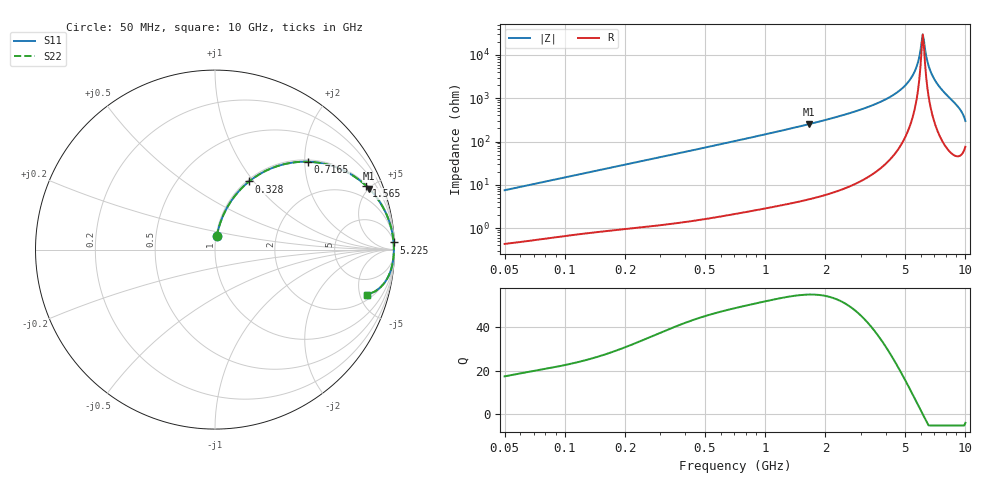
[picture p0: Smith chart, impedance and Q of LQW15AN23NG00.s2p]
!Murata Part Number: LQW15AN23NG00
!These Parameters are Measured in Series Mode Connection
!  o--[Z]--o
!Port1  Port2
!  o-------o
!Freq. Start=50[MHz] Stop=10[GHz], 401[Steps]
# Hz S RI R 50
!Freq.(Hz)	S 11(Real)	S 11(Imag)	S 21(Real)	S 21(Imag)	S 12(Real)	S 12(Imag)	S 22(Real)	S 22(Imag)
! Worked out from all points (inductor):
!   401 points, 50 MHz to 10 GHz, reference 50 ohm
!   read as one part in series: L = 23.7 nH near 51.34 MHz
!   highest Q = 54.6 at 1.651 GHz (marker M1), where L = 24.2 nH
!   self-resonance near 6.126 GHz
!   S11 on the Smith chart (normalised r, x): 50 MHz: 1.01, +0.15; 328 MHz: 1.02, +0.95; 716.5 MHz: 1.04, +2.08; 1.565 GHz: 1.09, +4.73; 5.225 GHz: 5, +50; 10 GHz: 2.51, -5.76
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5e7  0.00977 0.0737  0.9902 -0.0737  0.9902 -0.0737  0.00977 0.0737
1.214486e8  0.0374 0.1702  0.9626 -0.1702  0.9626 -0.1702  0.0374 0.1702
2.949953e8  0.1608 0.3541  0.8392 -0.3541  0.8392 -0.3541  0.1608 0.3541
3.279712e8  0.1899 0.3795  0.8101 -0.3795  0.8101 -0.3795  0.1899 0.3795
7.071068e8  0.5118 0.4896  0.4882 -0.4896  0.4882 -0.4896  0.5118 0.4896
7.165353e8  0.5184 0.4895  0.4816 -0.4895  0.4816 -0.4895  0.5184 0.4895
1.565451e9  0.8438 0.354  0.1562 -0.354  0.1562 -0.354  0.8438 0.354
1.65063e9  0.8585 0.3395  0.1415 -0.3395  0.1415 -0.3395  0.8585 0.3395
1.717543e9  0.8689 0.3285  0.1311 -0.3285  0.1311 -0.3285  0.8689 0.3285
2.917498e9  0.961 0.1831  0.039 -0.1831  0.039 -0.1831  0.961 0.1831
4.171863e9  0.9877 0.0939  0.0123 -0.0939  0.0123 -0.0939  0.9877 0.0939
5.225452e9  0.9952 0.0398  0.00482 -0.0398  0.00482 -0.0398  0.9952 0.0398
5.657692e9  0.9963 0.0203  0.00367 -0.0203  0.00367 -0.0203  0.9963 0.0203
6.045081e9  0.9967 0.0037  0.00334 -0.0037  0.00334 -0.0037  0.9967 0.0037
6.125686e9  0.9967 0.000302  0.00334 -0.000302  0.00334 -0.000302  0.9967 0.000302
6.290134e9  0.9966 -0.00658  0.00343 0.00658  0.00343 0.00658  0.9966 -0.00658
6.458996e9  0.9964 -0.0136  0.00363 0.0136  0.00363 0.0136  0.9964 -0.0136
6.632392e9  0.996 -0.0208  0.00395 0.0208  0.00395 0.0208  0.996 -0.0208
6.993273e9  0.995 -0.0357  0.005 0.0357  0.005 0.0357  0.995 -0.0357
7.672705e9  0.9914 -0.0646  0.00856 0.0646  0.00856 0.0646  0.9914 -0.0646
9.114482e9  0.9682 -0.1443  0.0318 0.1443  0.0318 0.1443  0.9682 -0.1443
1e10  0.8458 -0.253  0.1542 0.253  0.1542 0.253  0.8458 -0.253
